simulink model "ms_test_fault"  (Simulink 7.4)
settings: Solver=ode23t  StartTime=0.0  StopTime=15  RelTol=1e-5
undefined symbols (not defined in the file or in its folder): D1, Delta, dfilt, DiscIntNeverNeededParam
libraries: powerlib x47, simulink x12, powerlib_extras x8, dsparch4 x3
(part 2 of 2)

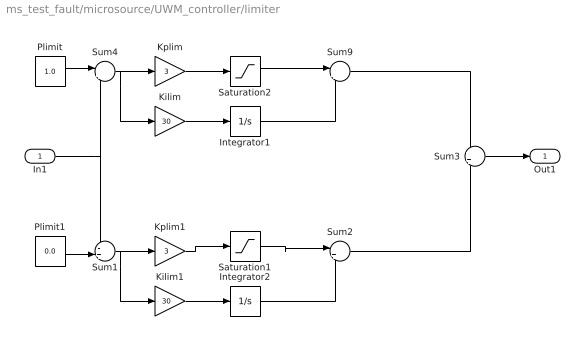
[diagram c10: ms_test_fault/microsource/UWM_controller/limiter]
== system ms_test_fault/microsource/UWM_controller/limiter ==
  In1 : Inport
  Integrator1 : Integrator  LimitOutput=on  UpperSaturationLimit=0  LowerSaturationLimit=-pi  ZeroCross=off
  Integrator2 : Integrator  LimitOutput=on  UpperSaturationLimit=pi  LowerSaturationLimit=0  ZeroCross=off
  Kilim : Gain  Gain=30  ParameterDataType=sfix(16)  ParameterScaling=2^0  OutDataType=sfix(16)  OutScaling=2^0
  Kilim1 : Gain  Gain=30  ParameterDataType=sfix(16)  ParameterScaling=2^0  OutDataType=sfix(16)  OutScaling=2^0
  Kplim : Gain  Gain=3  ParameterDataType=sfix(16)  ParameterScaling=2^0  OutDataType=sfix(16)  OutScaling=2^0
  Kplim1 : Gain  Gain=3  ParameterDataType=sfix(16)  ParameterScaling=2^0  OutDataType=sfix(16)  OutScaling=2^0
  Plimit : Constant  Value=1.0  OutDataType=sfix(16)  OutScaling=2^0
  Plimit1 : Constant  Value=0.0  OutDataType=sfix(16)  OutScaling=2^0
  Saturation1 : Saturate  UpperLimit=pi  LowerLimit=0  OutDataType=fixdt(1, 16)  OutScaling=2^0
  Saturation2 : Saturate  UpperLimit=0  LowerLimit=-pi  OutDataType=fixdt(1, 16)  OutScaling=2^0
  Sum1 : Sum  Inputs=-+|  OutDataType=sfix(16)  OutScaling=2^0
  Sum2 : Sum  Inputs=|++  OutDataType=sfix(16)  OutScaling=2^0
  Sum3 : Sum  OutDataType=sfix(16)  OutScaling=2^0
  Sum4 : Sum  Inputs=|+-  OutDataType=sfix(16)  OutScaling=2^0
  Sum9 : Sum  Inputs=|++  OutDataType=sfix(16)  OutScaling=2^0
  Out1 : Outport
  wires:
  Sum3/1 -> Out1/1
  Plimit1/1 -> Sum1/2
  Integrator2/1 -> Sum2/2
  Kilim1/1 -> Integrator2/1
  Sum1/1 -> Kilim1/1, Kplim1/1
  In1/1 -> Sum1/1, Sum4/2
  Integrator1/1 -> Sum9/2
  Kilim/1 -> Integrator1/1
  Sum4/1 -> Kilim/1, Kplim/1
  Plimit/1 -> Sum4/1
  Kplim1/1 -> Saturation1/1
  Saturation1/1 -> Sum2/1
  Kplim/1 -> Saturation2/1
  Saturation2/1 -> Sum9/1
  Sum9/1 -> Sum3/1
  Sum2/1 -> Sum3/2

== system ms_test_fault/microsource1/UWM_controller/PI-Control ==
  In1 : Inport
  Gain : Gain  Gain=.01  ParameterDataType=sfix(16)  ParameterScaling=2^0  OutDataType=sfix(16)  OutScaling=2^0
  Gain1 : Gain  Gain=5  ParameterDataType=sfix(16)  ParameterScaling=2^0  OutDataType=sfix(16)  OutScaling=2^0
  Gain2 : Gain  Gain=750  ParameterDataType=sfix(16)  ParameterScaling=2^0  OutDataType=sfix(16)  OutScaling=2^0
  Integrator1 : Integrator  LimitOutput=on  UpperSaturationLimit=100  LowerSaturationLimit=-100  ZeroCross=off
  Sum4 : Sum  Inputs=|++  OutDataType=sfix(16)  OutScaling=2^0
  Out1 : Outport
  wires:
  Gain/1 -> Sum4/1
  Integrator1/1 -> Sum4/2
  In1/1 -> Gain1/1, Gain/1
  Gain1/1 -> Integrator1/1
  Sum4/1 -> Gain2/1
  Gain2/1 -> Out1/1

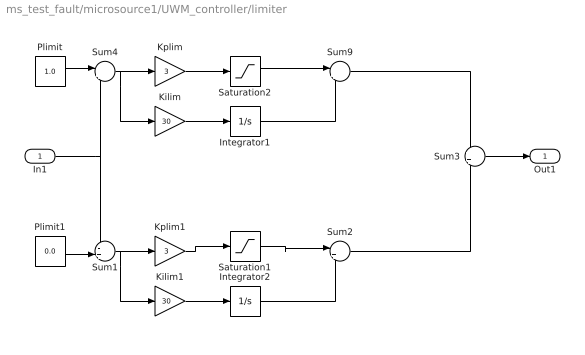
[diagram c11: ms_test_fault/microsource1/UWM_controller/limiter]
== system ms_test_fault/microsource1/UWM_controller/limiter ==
  In1 : Inport
  Integrator1 : Integrator  LimitOutput=on  UpperSaturationLimit=0  LowerSaturationLimit=-pi  ZeroCross=off
  Integrator2 : Integrator  LimitOutput=on  UpperSaturationLimit=pi  LowerSaturationLimit=0  ZeroCross=off
  Kilim : Gain  Gain=30  ParameterDataType=sfix(16)  ParameterScaling=2^0  OutDataType=sfix(16)  OutScaling=2^0
  Kilim1 : Gain  Gain=30  ParameterDataType=sfix(16)  ParameterScaling=2^0  OutDataType=sfix(16)  OutScaling=2^0
  Kplim : Gain  Gain=3  ParameterDataType=sfix(16)  ParameterScaling=2^0  OutDataType=sfix(16)  OutScaling=2^0
  Kplim1 : Gain  Gain=3  ParameterDataType=sfix(16)  ParameterScaling=2^0  OutDataType=sfix(16)  OutScaling=2^0
  Plimit : Constant  Value=1.0  OutDataType=sfix(16)  OutScaling=2^0
  Plimit1 : Constant  Value=0.0  OutDataType=sfix(16)  OutScaling=2^0
  Saturation1 : Saturate  UpperLimit=pi  LowerLimit=0  OutDataType=fixdt(1, 16)  OutScaling=2^0
  Saturation2 : Saturate  UpperLimit=0  LowerLimit=-pi  OutDataType=fixdt(1, 16)  OutScaling=2^0
  Sum1 : Sum  Inputs=-+|  OutDataType=sfix(16)  OutScaling=2^0
  Sum2 : Sum  Inputs=|++  OutDataType=sfix(16)  OutScaling=2^0
  Sum3 : Sum  OutDataType=sfix(16)  OutScaling=2^0
  Sum4 : Sum  Inputs=|+-  OutDataType=sfix(16)  OutScaling=2^0
  Sum9 : Sum  Inputs=|++  OutDataType=sfix(16)  OutScaling=2^0
  Out1 : Outport
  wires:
  Sum3/1 -> Out1/1
  Plimit1/1 -> Sum1/2
  Integrator2/1 -> Sum2/2
  Kilim1/1 -> Integrator2/1
  Sum1/1 -> Kilim1/1, Kplim1/1
  In1/1 -> Sum1/1, Sum4/2
  Integrator1/1 -> Sum9/2
  Kilim/1 -> Integrator1/1
  Sum4/1 -> Kilim/1, Kplim/1
  Plimit/1 -> Sum4/1
  Kplim1/1 -> Saturation1/1
  Saturation1/1 -> Sum2/1
  Kplim/1 -> Saturation2/1
  Saturation2/1 -> Sum9/1
  Sum9/1 -> Sum3/1
  Sum2/1 -> Sum3/2

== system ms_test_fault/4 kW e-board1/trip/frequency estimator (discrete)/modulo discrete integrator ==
  In1 : Inport
  Abs : Abs
  Constant1 : Constant  OutDataType=sfix(16)  OutScaling=2^0
  Discrete-Time Integrator : DiscreteIntegrator  ExternalReset=rising  InitialConditionSource=external  SampleTime=dt  OutDataType=fixdt(1, 16)  OutScaling=2^0  UpperSaturationLimit=100  LowerSaturationLimit=-100  ShowStatePort=on  ICPrevOutput=DiscIntNeverNeededParam  ICPrevScaledInput=DiscIntNeverNeededParam
  Gain1 : Gain  Gain=1+.0001  ParameterDataType=sfix(16)  ParameterScaling=2^0  OutDataType=sfix(16)  OutScaling=2^0
  IC : InitialCondition  Value=0
  Math Function : Math  Operator=rem  OutDataType=sfix(16)  OutScaling=2^0
  Relational Operator : RelationalOperator
  Out1 : Outport
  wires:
  Relational Operator/1 -> Discrete-Time Integrator/2
  Discrete-Time Integrator/State -> Gain1/1
  Gain1/1 -> Abs/1
  Constant1/1 -> Relational Operator/2, Math Function/2
  Abs/1 -> Relational Operator/1, Math Function/1
  In1/1 -> Discrete-Time Integrator/1
  Discrete-Time Integrator/1 -> Out1/1
  IC/1 -> Discrete-Time Integrator/3
  Math Function/1 -> IC/1

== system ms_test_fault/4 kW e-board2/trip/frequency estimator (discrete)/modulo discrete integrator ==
  In1 : Inport
  Abs : Abs
  Constant1 : Constant  OutDataType=sfix(16)  OutScaling=2^0
  Discrete-Time Integrator : DiscreteIntegrator  ExternalReset=rising  InitialConditionSource=external  SampleTime=dt  OutDataType=fixdt(1, 16)  OutScaling=2^0  UpperSaturationLimit=100  LowerSaturationLimit=-100  ShowStatePort=on  ICPrevOutput=DiscIntNeverNeededParam  ICPrevScaledInput=DiscIntNeverNeededParam
  Gain1 : Gain  Gain=1+.0001  ParameterDataType=sfix(16)  ParameterScaling=2^0  OutDataType=sfix(16)  OutScaling=2^0
  IC : InitialCondition  Value=0
  Math Function : Math  Operator=rem  OutDataType=sfix(16)  OutScaling=2^0
  Relational Operator : RelationalOperator
  Out1 : Outport
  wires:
  Relational Operator/1 -> Discrete-Time Integrator/2
  Discrete-Time Integrator/State -> Gain1/1
  Gain1/1 -> Abs/1
  Constant1/1 -> Relational Operator/2, Math Function/2
  Abs/1 -> Relational Operator/1, Math Function/1
  In1/1 -> Discrete-Time Integrator/1
  Discrete-Time Integrator/1 -> Out1/1
  IC/1 -> Discrete-Time Integrator/3
  Math Function/1 -> IC/1
